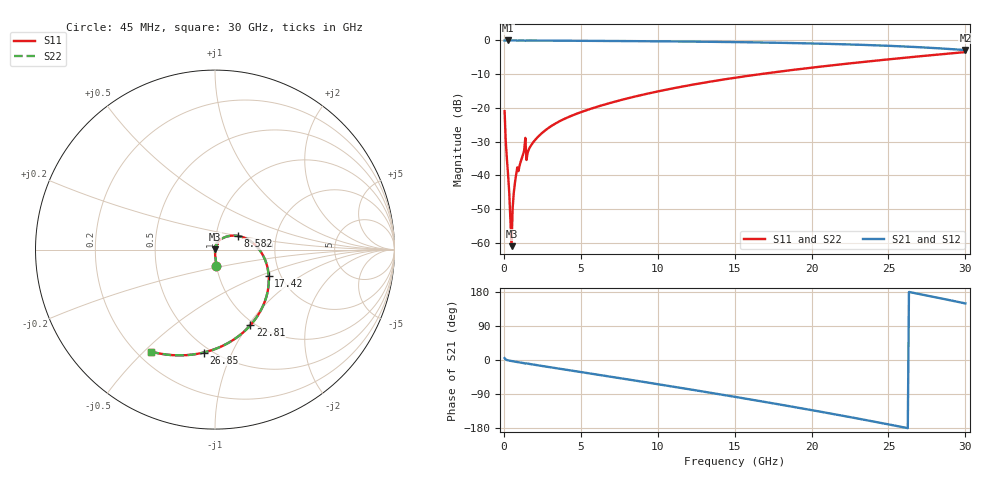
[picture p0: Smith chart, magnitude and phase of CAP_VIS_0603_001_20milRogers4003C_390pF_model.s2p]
! S-parameter model data by Modelithics Inc.  support@modelithics.com  813-866-6335  Tampa FL USA
! S-Parameter data specifications:
! Substrate: 20-mil Rogers 4003C, substrate thickness, H=0.508mm, Dielectric constant, Er=3.75
! PCB Mounting Pad Footprint: Pad width, PadW=0.90mm , Pad length, PadL=1.00mm , Pad gap, PadG (edge-to-edge)=1.00mm , Reference planes=3.0mm apart
! Created Wed Nov 18 13:34:26 2015
# hz S ma R 50
! 2 Port Network Data from SP1.SP block
! freq  magS11  angS11  magS21  angS21  magS12  angS12  magS22  angS22
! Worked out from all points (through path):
!   401 points, 45 MHz to 30 GHz, reference 50 ohm
!   highest |S21| = 0.00 dB at 269.7 MHz (marker M1); lowest = -2.9 dB at 30 GHz (marker M2)
!   group delay of S21, straight-line fit = 19.3 ps
!   lowest |S11| = -61.0 dB at 494.3 MHz (marker M3), VSWR 1.00, Z = 50 + j0.0736 ohm
!   |S11| at or under -10 dB: start of sweep to 16.66 GHz
!   |S22| runs from -61.0 to -3.5 dB; largest |S21 - S12| = 0
!   S11 on the Smith chart (normalised r, x): 45 MHz: 1.00, -0.18; 8.582 GHz: 1.27, +0.20; 17.42 GHz: 1.73, -0.57; 22.81 GHz: 0.95, -1.03; 26.85 GHz: 0.46, -0.79; 30 GHz: 0.25, -0.52
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4.5e7  0.0893 -85.0  0.9958 4.9  0.9958 4.9  0.0893 -85.0
1.94775e8  0.01739 -89.0  0.9995 -0.1  0.9995 -0.1  0.01739 -89.0
2.696625e8  0.01024 -88.9  0.9996 -0.9  0.9996 -0.9  0.01024 -88.9
3.4455e8  0.005602 -87.5  0.9996 -1.5  0.9996 -1.5  0.005602 -87.5
4.94325e8  0.0008879 55.9  0.9995 -2.7  0.9995 -2.7  0.0008879 55.9
5.692125e8  0.003299 78.1  0.9994 -3.3  0.9994 -3.3  0.003299 78.1
7.189875e8  0.007816 81.2  0.9993 -4.3  0.9993 -4.3  0.007816 81.2
7.93875e8  0.01025 80.4  0.999 -4.9  0.999 -4.9  0.01025 80.4
1.2432e9  0.02029 79.4  0.9987 -7.9  0.9987 -7.9  0.02029 79.4
1.617638e9  0.02415 77.2  0.9984 -10.1  0.9984 -10.1  0.02415 77.2
2.066962e9  0.03423 74.2  0.9976 -13.1  0.9976 -13.1  0.03423 74.2
2.965612e9  0.05162 67.1  0.9948 -18.9  0.9948 -18.9  0.05162 67.1
5.062462e9  0.08728 51.9  0.9868 -32.2  0.9868 -32.2  0.08728 51.9
8.582175e9  0.1483 30.9  0.9764 -54.6  0.9764 -54.6  0.1483 30.9
1.007992e10  0.1768 21.7  0.9712 -64.3  0.9712 -64.3  0.1768 21.7
1.50225e10  0.2796 -10.0  0.9454 -97.2  0.9454 -97.2  0.2796 -10.0
1.74189e10  0.3335 -26.2  0.9272 -113.8  0.9272 -113.8  0.3335 -26.2
2.003996e10  0.3954 -44.6  0.9019 -132.5  0.9019 -132.5  0.3954 -44.6
2.28108e10  0.4652 -64.9  0.8674 -153.0  0.8674 -153.0  0.4652 -64.9
2.505742e10  0.5258 -82.1  0.8317 -170.3  0.8317 -170.3  0.5258 -82.1
2.685472e10  0.577 -96.3  0.7968 175.3  0.7968 175.3  0.577 -96.3
3e10  0.6714 -122.2  0.7191 149.3  0.7191 149.3  0.6714 -122.2
